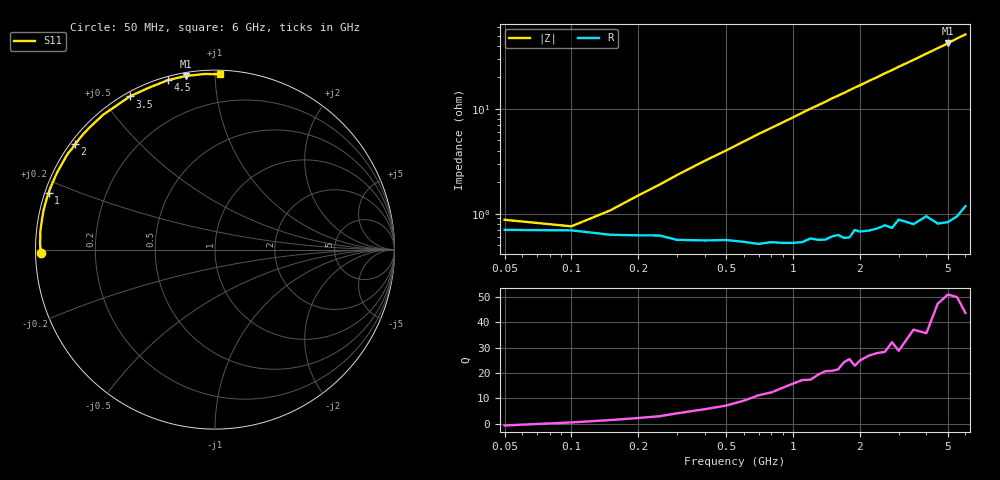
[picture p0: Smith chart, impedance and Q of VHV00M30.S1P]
! Infineon Technologies  Discrete & RF Semiconductors
! BB 814
! Si Tuning Diode in SOT23
! VR =
! S-Parameters:  July  1999
# GHz  S  MA  R  50
!  f  S11
! GHz  MAG  ANG
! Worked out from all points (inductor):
!   34 points, 50 MHz to 6 GHz, reference 50 ohm
!   read as one part to ground: L = 1.25 nH near 300 MHz
!   highest Q = 49.9 at 5 GHz (marker M1), where L = 1.34 nH
!   S11 on the Smith chart (normalised r, x): 50 MHz: 0.01, -0.01; 1 GHz: 0.01, +0.17; 2 GHz: 0.01, +0.33; 3.5 GHz: 0.02, +0.59; 4.5 GHz: 0.02, +0.76; 6 GHz: 0.02, +1.03
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0.05  0.9724 -178.8
0.1  0.9727 179.3
0.15  0.9752 178.0
0.2  0.9755 176.9
0.3  0.9778 174.8
0.4  0.9781 172.8
0.6  0.9789 168.9
0.8  0.9792 165.0
1  0.9797 161.2
1.2  0.978 157.3
1.4  0.9788 153.7
1.5  0.9775 151.7
1.6  0.9769 150.0
1.7  0.9785 148.3
1.8  0.9785 146.4
1.9  0.9749 144.6
2  0.976 143.0
2.2  0.976 139.4
2.4  0.9754 136.2
2.6  0.9744 132.7
2.8  0.9763 129.7
3  0.9724 126.4
3.5  0.9767 119.1
4  0.9743 112.0
4.5  0.9798 105.5
5  0.9808 99.6
5.5  0.9802 93.4
6  0.9774 88.4
